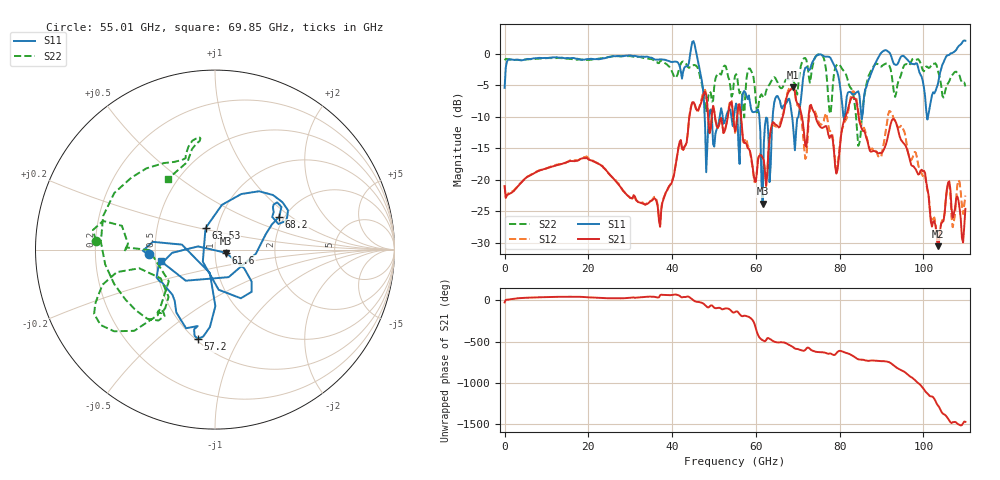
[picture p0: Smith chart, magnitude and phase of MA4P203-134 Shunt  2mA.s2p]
!Keysight Technologies,N5247B,US61255204,A.15.70.20
!Date: Friday, October 21, 2022 15:21:26
!Correction: S11(C  4-Port  )
!S31(C  4-Port  )
!S13(C  4-Port  )
!S33(C  4-Port  )
!S2P File: Measurements: S11, S31, S13, S33:
# Hz S  dB  R 50
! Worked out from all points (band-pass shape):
!   401 points, 10 MHz to 110 GHz, reference 50 ohm
!   highest |S21| = -5.31 dB at 68.75 GHz (marker M1); lowest = -30.6 dB at 103.4 GHz (marker M2)
!   |S21| within 3 dB of the highest: 66.92 GHz to 70.39 GHz (3.471 GHz wide, 5.06 % of centre); 82.15 GHz to 84.18 GHz (2.028 GHz wide, 2.44 % of centre)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
!   lowest |S11| = -23.8 dB at 61.6 GHz (marker M3), VSWR 1.14, Z = 56.6 - j2.07 ohm
!   |S11| at or under -10 dB: 49.45 GHz to 51.36 GHz (1.916 GHz wide, 3.8 % of centre); 60.82 GHz to 64.01 GHz (3.192 GHz wide, 5.12 % of centre); 68.64 GHz to 70.15 GHz (1.512 GHz wide, 2.18 % of centre)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
!   |S22| runs from -14.6 to 0.0 dB; largest |S21 - S12| = 0.17
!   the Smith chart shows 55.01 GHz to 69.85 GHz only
!   S11 on the Smith chart (normalised r, x): 55.01 GHz: 0.46, -0.03; 57.2 GHz: 0.51, -0.69; 61.6 GHz: 1.13, -0.04; 63.53 GHz: 0.88, +0.21; 68.2 GHz: 1.88, +0.82; 69.85 GHz: 0.53, -0.08
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1e7  -5.42 -177.0  -21.03 -25.7  -20.91 -25.7  -1.02 -177.1
1.843332e10  -0.96 145.8  -16.63 40.9  -16.61 40.7  -0.92 145.4
3.685665e10  -0.93 154.6  -26.48 35.9  -26.13 36.4  -1.48 154.3
4.51059e10  2.00 85.2  -7.69 -0.9  -7.64 -3.2  -1.81 115.4
4.813062e10  -18.81 59.8  -6.58 -71.5  -6.41 -72.0  -9.26 113.3
5.5005e10  -8.63 -175.8  -12.30 -142.5  -12.55 -144.3  -3.53 175.7
5.72048e10  -5.91 -100.9  -14.18 173.8  -14.03 -177.8  -10.11 -145.5
6.16044e10  -23.79 -16.4  -16.54 -122.8  -16.63 -120.9  -6.75 -132.9
6.352922e10  -17.68 113.9  -12.05 -113.6  -12.41 -110.7  -4.53 -161.2
6.82038e10  -7.91 27.1  -5.76 173.4  -5.30 170.1  -4.01 97.8
6.875375e10  -10.58 17.0  -5.31 157.8  -5.04 153.7  -4.28 98.1
6.985365e10  -10.22 -167.9  -7.89 131.4  -8.16 130.8  -6.50 123.6
7.342832e10  -1.39 178.3  -8.70 112.2  -8.68 107.4  -2.25 156.3
7.645305e10  -0.45 -165.6  -11.54 87.2  -9.93 118.7  -1.30 148.0
7.947778e10  -3.03 -147.6  -18.43 96.1  -17.65 94.5  -1.68 -137.2
8.415235e10  -6.07 -38.9  -8.19 13.0  -7.72 17.7  -12.33 -170.3
8.745205e10  -3.20 49.8  -15.56 -8.5  -15.19 5.0  -2.70 53.5
9.185165e10  0.20 88.6  -12.04 -30.3  -9.08 -23.0  -1.92 76.1
9.817608e10  -1.50 175.9  -18.39 104.7  -15.72 103.6  -0.96 -174.5
1.034006e11  -4.89 -37.6  -30.56 170.0  -30.52 174.3  -2.60 -110.7
1.069753e11  0.16 10.4  -26.05 -34.5  -27.54 -38.5  -3.29 -23.5
1.1e11  2.07 46.1  -24.63 -29.6  -22.53 -28.0  -5.19 10.3
